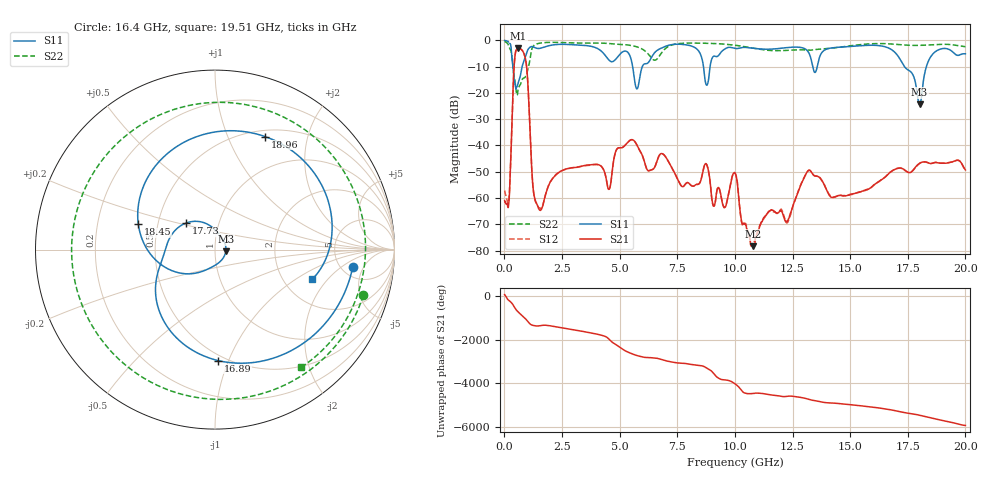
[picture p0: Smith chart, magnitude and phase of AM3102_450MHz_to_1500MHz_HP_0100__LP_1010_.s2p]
!Agilent Technologies,E8364B,MY43040894,A.07.50.67
!Agilent E8364B: A.07.50.67
!Date: Thursday, January 11, 2018 05:37:42
!Correction: S11(Full 2 Port(1,2))
!S21(Full 2 Port(1,2))
!S12(Full 2 Port(1,2))
!S22(Full 2 Port(1,2))
!S2P File: Measurements: S11, S21, S12, S22:
# Hz S  dB  R 50
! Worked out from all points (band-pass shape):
!   1601 points, 10 MHz to 20 GHz, reference 50 ohm
!   highest |S21| = -3.09 dB at 609.7 MHz (marker M1); lowest = -78.3 dB at 10.78 GHz (marker M2)
!   |S21| within 3 dB of the highest: 457.9 MHz to 887.2 MHz (429.4 MHz wide, 63.8 % of centre)
!   lowest |S11| = -24.3 dB at 18.01 GHz (marker M3), VSWR 1.13, Z = 56.4 - j1.13 ohm
!   |S11| at or under -10 dB: 365.6 MHz to 769.7 MHz (404.1 MHz wide, 71.2 % of centre); 5.565 GHz to 5.984 GHz (419.8 MHz wide, 7.27 % of centre); 17.36 GHz to 18.31 GHz (950.9 MHz wide, 5.33 % of centre)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
!   |S22| runs from -20.9 to -0.5 dB; largest |S21 - S12| = 0.0026
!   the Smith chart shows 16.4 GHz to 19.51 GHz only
!   S11 on the Smith chart (normalised r, x): 16.4 GHz: 6.31, -3.07; 16.89 GHz: 0.46, -0.92; 17.73 GHz: 0.69, +0.22; 18.45 GHz: 0.39, +0.14; 18.96 GHz: 0.58, +1.38; 19.51 GHz: 2.87, -1.40
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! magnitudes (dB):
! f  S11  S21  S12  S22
! 10 MHz  -0.1  -61.0  -57.2  -0.5
! 184.9 MHz  -0.6  -62.6  -61.5  -2.0
! 434.8 MHz  -15.0  -8.3  -8.3  -14.3
! 609.7 MHz  -15.7  -3.1  -3.1  -18.2
! 934.5 MHz  -5.5  -8.0  -8.0  -13.5
! 1.247 GHz  -2.5  -56.4  -56.5  -2.3
! 1.459 GHz  -3.1  -63.2  -63.2  -1.2
! 3.346 GHz  -1.9  -47.9  -48.0  -1.1
! 5.745 GHz  -18.5  -39.8  -39.8  -2.5
! 6.682 GHz  -3.5  -44.4  -44.5  -6.5
! 10.01 GHz  -3.1  -50.5  -50.5  -1.9
! 10.78 GHz  -3.0  -78.3  -77.8  -3.0
! 13.34 GHz  -8.6  -50.5  -50.4  -3.7
! 16.4 GHz  -2.2  -52.8  -52.8  -1.3
! 16.68 GHz  -3.0  -50.7  -50.7  -1.4
! 16.89 GHz  -4.2  -49.3  -49.3  -1.5
! 17.73 GHz  -13.2  -49.5  -49.5  -1.9
! 18.01 GHz  -24.3  -46.8  -46.9  -1.9
! 18.45 GHz  -6.9  -46.9  -46.8  -1.8
! 18.96 GHz  -3.2  -46.8  -46.8  -1.5
! 19.51 GHz  -4.9  -46.0  -46.1  -1.8
! 20 GHz  -5.1  -49.3  -49.5  -2.4
